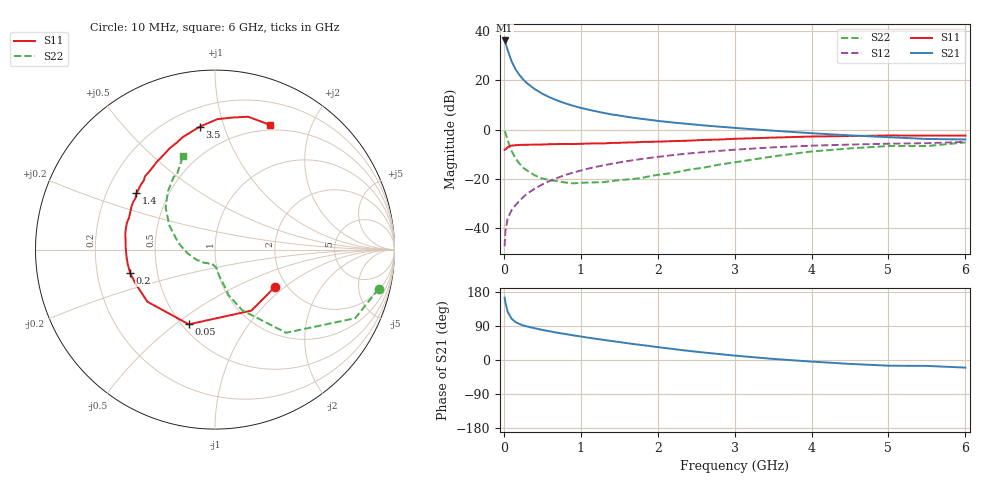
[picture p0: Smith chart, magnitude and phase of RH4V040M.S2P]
! SIEMENS Small Signal Semiconductors
! BFR106
! Si NPN RF Bipolar Junction Transistor in SOT23
! VCE = 4 V  IC = 40 mA
! Common Emitter S-Parameters:  August  1996
# GHz  S  MA  R  50
!  f  S11  S21  S12  S22
! GHz  MAG  ANG  MAG  ANG  MAG  ANG  MAG  ANG
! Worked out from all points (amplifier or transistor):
!   36 points, 10 MHz to 6 GHz, reference 50 ohm
!   highest |S21| = 36.3 dB at 10 MHz (marker M1)
!   |S21| within 3 dB of that: start of sweep to 40.7 MHz
!   unconditionally stable (mu >= 1): 269.6 MHz to 2.313 GHz
!   at 250 MHz: K = 0.99, MSG = 24.0 dB, |S12| = -27.5 dB
!   at 1.4 GHz: K = 1.06, MAG = 8.6 dB, |S12| = -13.9 dB
!   at 6 GHz: K = 0.99, MSG = 0.5 dB, |S12| = -5.0 dB
!   S11 on the Smith chart (normalised r, x): 10 MHz: 1.74, -0.85; 50 MHz: 0.54, -0.56; 200 MHz: 0.35, -0.12; 1.4 GHz: 0.33, +0.29; 3.5 GHz: 0.32, +0.83; 6 GHz: 0.44, +1.44
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0.01  0.3935 -31.7  65.03 164.7  0.0043 81.6  0.9374 -13.5
0.02  0.3959 -59.2  59.26 152.2  0.0086 71.9  0.8694 -26.1
0.05  0.4411 -109.3  41.1 127.2  0.0158 59.6  0.6094 -49.5
0.1  0.4758 -142.4  24.67 109.2  0.023 59.3  0.3707 -65.8
0.15  0.4821 -157.3  17.14 100.3  0.029 62.2  0.2651 -73.4
0.2  0.4905 -164.5  13.13 95.3  0.0357 64.9  0.2076 -75.6
0.25  0.4926 -170.2  10.54 91.3  0.0424 67.2  0.1692 -78.8
0.3  0.4941 -174.2  8.836 88.6  0.0498 68.7  0.1488 -80.8
0.4  0.4974 179.2  6.707 83.9  0.063 70.3  0.1185 -83.8
0.5  0.4998 174.9  5.385 79.5  0.0772 70.7  0.1018 -86.1
0.6  0.5072 170.3  4.513 75.6  0.0916 70.3  0.0944 -88.9
0.7  0.5105 166.5  3.897 71.8  0.1057 69.8  0.0898 -93.2
0.9  0.5109 159.6  3.064 65.2  0.1345 67.8  0.0814 -100.2
1.1  0.5227 153.0  2.551 58.8  0.1621 65.6  0.0848 -110.0
1.4  0.5382 144.4  2.047 50.3  0.2027 61.5  0.0902 -123.8
1.7  0.5525 136.0  1.734 41.7  0.2422 57.4  0.1001 -139.9
2.2  0.5859 123.8  1.398 29.1  0.3048 49.8  0.1327 -162.5
2.8  0.6313 110.0  1.153 15.7  0.3713 40.5  0.1951 172.7
3.5  0.6908 96.9  0.955 2.9  0.4383 30.0  0.2869 152.3
4.5  0.7426 82.3  0.766 -10.3  0.498 15.3  0.4175 128.9
5.5  0.7582 69.9  0.648 -15.6  0.5321 5.6  0.4656 117.3
6  0.7588 66.1  0.634 -20.1  0.5643 -1.5  0.5522 108.8
